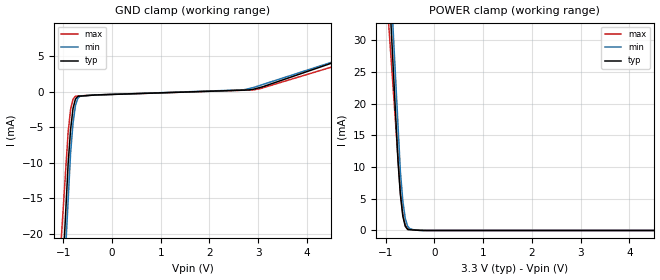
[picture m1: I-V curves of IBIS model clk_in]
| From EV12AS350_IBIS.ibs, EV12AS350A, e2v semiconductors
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[Model] clk_in
Model_type Input
Vinl = 1.54200V
Vinh = 1.85800V
C_comp 430.000fF 428.000fF 432.000fF
| variable typ   min   max
[Voltage Range] 3.30000V 3.20000V 3.40000V
[POWER Clamp Reference] 3.30000V 3.20000V 3.40000V
[GND Clamp Reference] 0.00000V 0.00000V 0.00000V
[Temperature Range]   25   110   -40
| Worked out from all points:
|   GND clamp passes 1 mA (typ) near -0.75 V on its own axis
|   POWER clamp passes 1 mA (typ) near -0.61 V on its own axis
[GND Clamp]
-3.3V     -337.7mA   -335.5mA   -261.5mA
-900mV    -10.12mA   -15.3mA    -5.681mA
-850mV    -5.342mA   -8.624mA   -2.489mA
-800mV    -2.339mA   -4.428mA   -1.027mA
-750mV    -1.012mA   -1.905mA   -607.7uA
-700mV    -617.5uA   -877.4uA   -585.1uA
-650mV    -591.9uA   -589.9uA   -562.5uA
2.7V      247.6uA    288.3uA    235.6uA
2.9V      364.8uA    610.6uA    279.5uA
3.05V     645.1uA    944uA      477.5uA
6.6V      8.983mA    8.834mA    7.848mA
[POWER Clamp]
-3.3V     394mA      398.9mA    293.2mA
-800mV    18.57mA    24.24mA    17.07mA
-750mV    11.06mA    16.75mA    11.55mA
-700mV    5.661mA    9.255mA    6.025mA
-650mV    2.264mA    4.634mA    2.543mA
-600mV    664.1uA    1.882mA    843.9uA
-550mV    137.7uA    649.9uA    303.4uA
-500mV    112.7uA    248uA      211.8uA
-275mV    0A         10.63uA    43.71uA
6.6V      0A         0A         0A
